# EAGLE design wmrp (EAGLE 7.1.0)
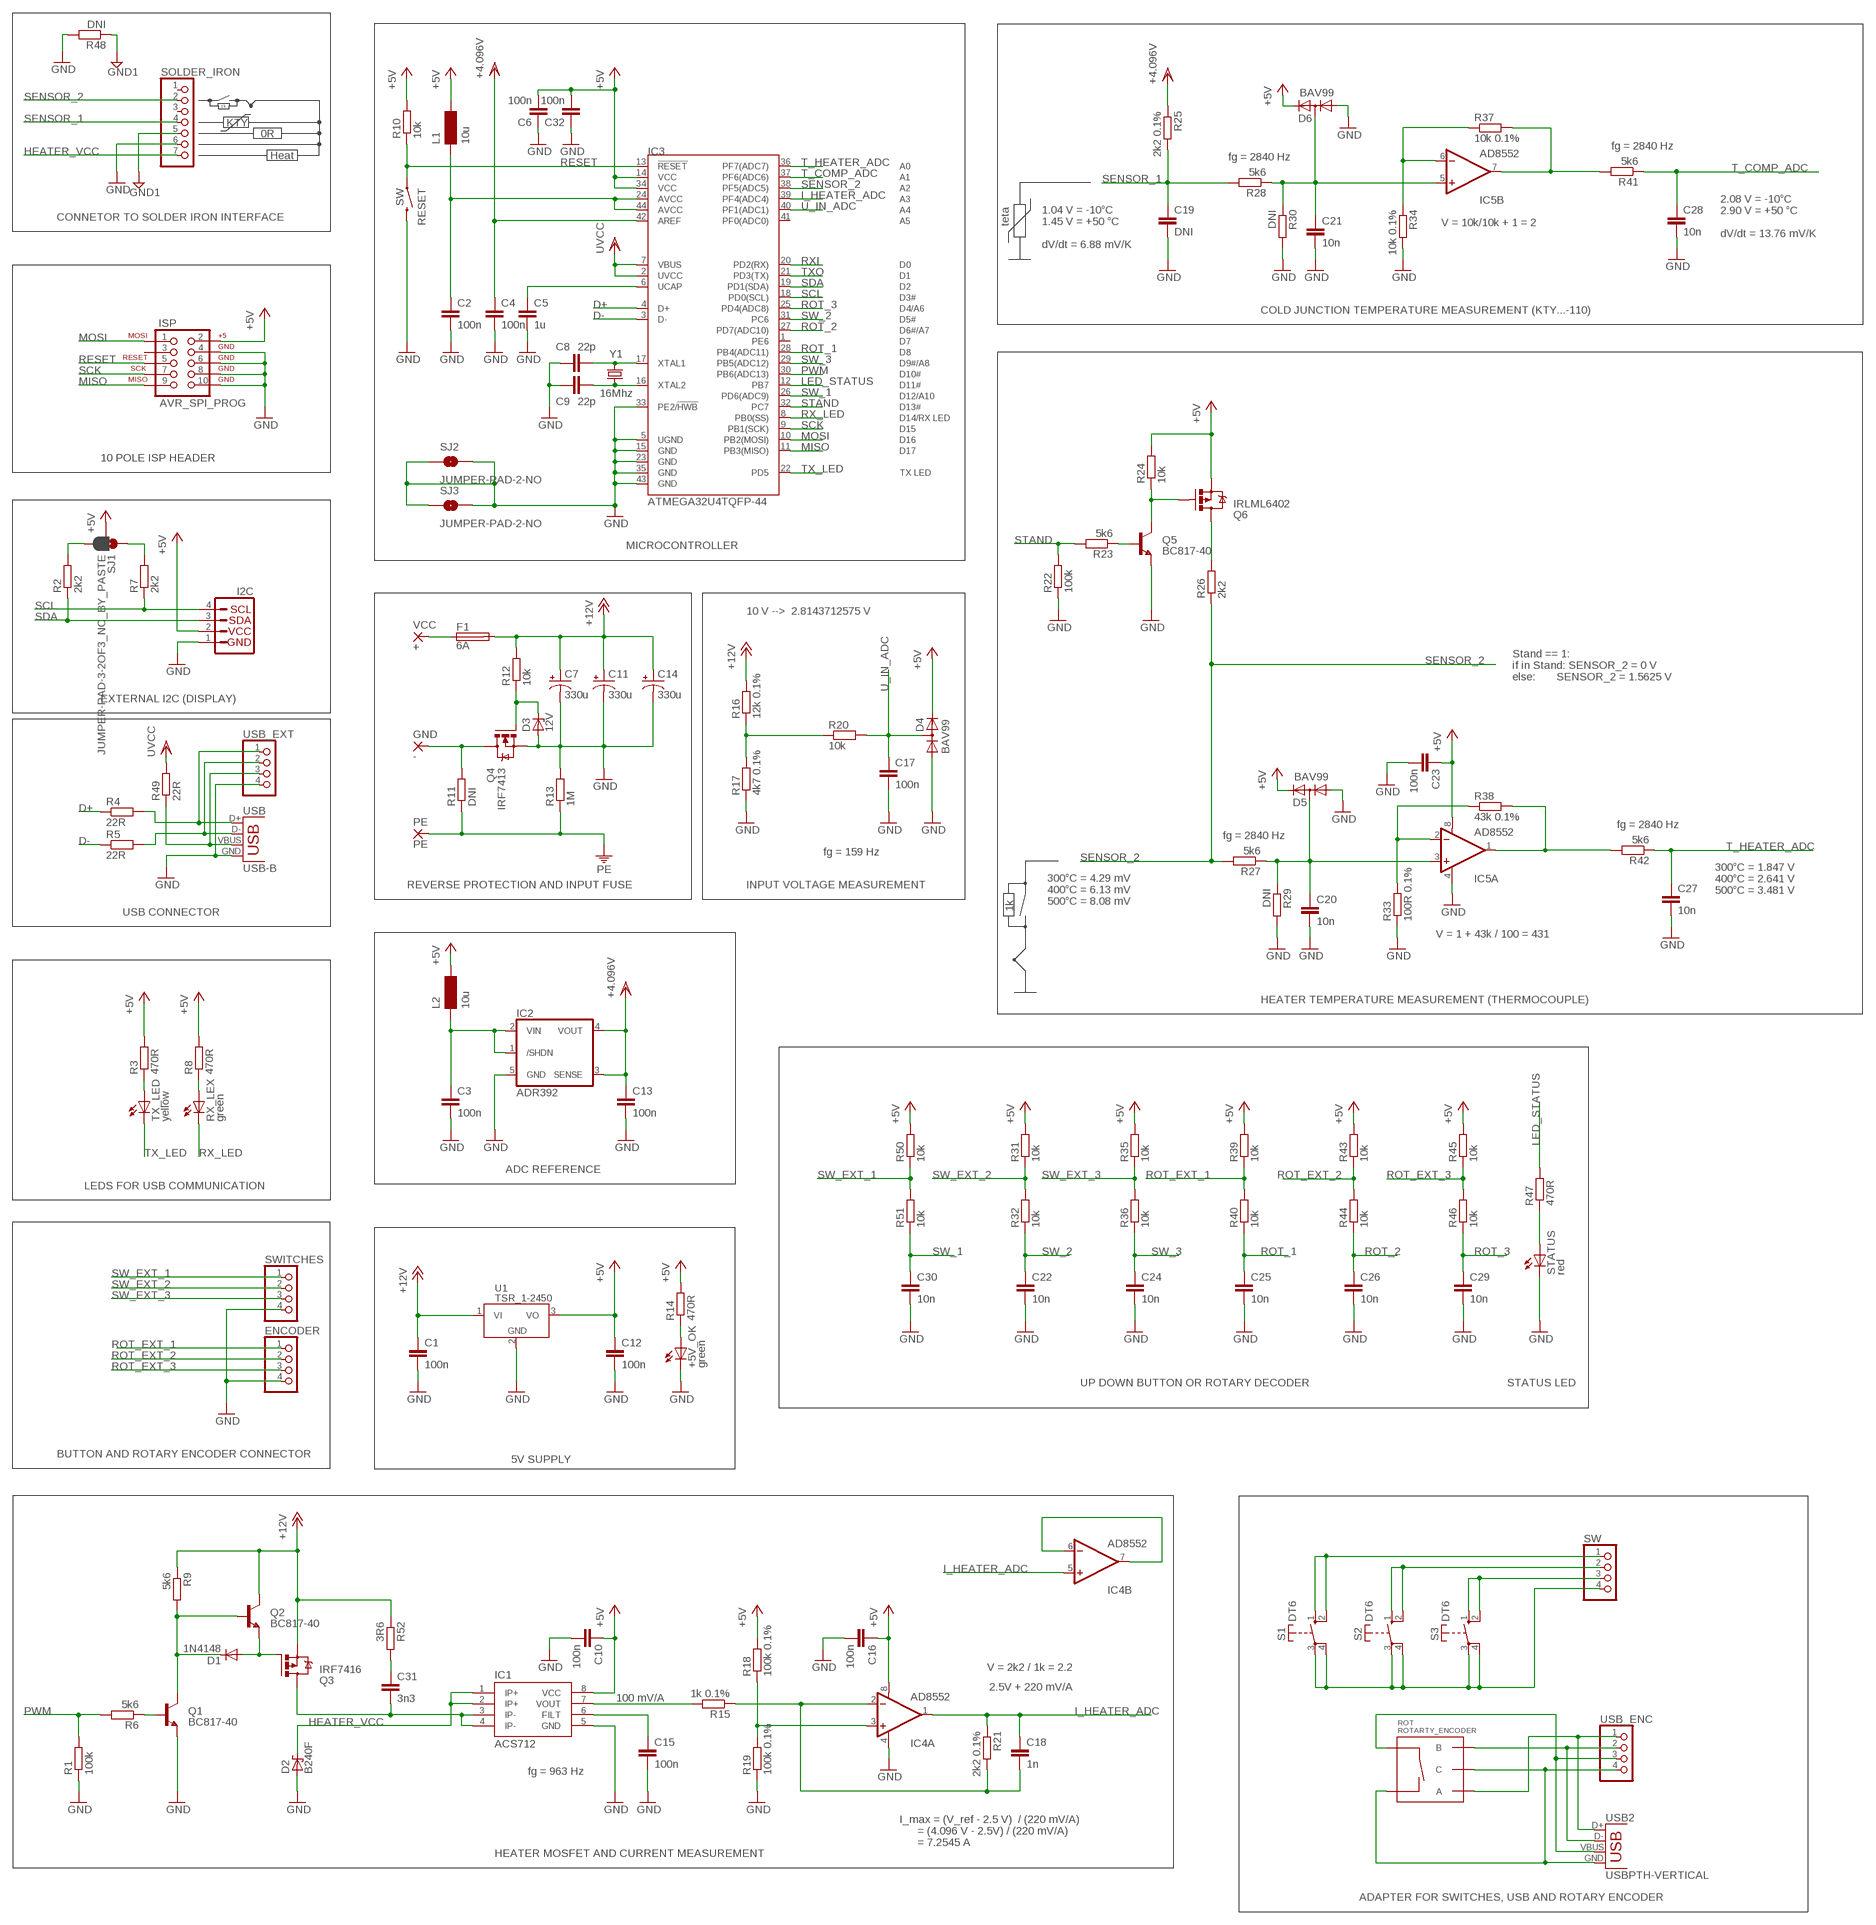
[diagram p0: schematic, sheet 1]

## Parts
+5V_OK  green  LEDCHIPLED_1206  [CHIPLED_1206]
C1  100n  C-EUC1206  [C1206]
C2  100n  C-EUC1206  [C1206]
C3  100n  C-EUC1206  [C1206]
C4  100n  C-EUC1206  [C1206]
C5  1u  C-EUC1206  [C1206]
C6  100n  C-EUC1206  [C1206]
C7  330u  CAP_POLPTH4  [CPOL-RADIAL-1000UF-25V]
C8  22p  C-EUC1206  [C1206]
C9  22p  C-EUC1206  [C1206]
C10  100n  C-EUC1206  [C1206]
C11  330u  CAP_POLPTH4  [CPOL-RADIAL-1000UF-25V]
C12  100n  C-EUC1206  [C1206]
C13  100n  C-EUC1206  [C1206]
C14  330u  CAP_POLPTH4  [CPOL-RADIAL-1000UF-25V]
C15  100n  C-EUC1206  [C1206]
C16  100n  C-EUC1206  [C1206]
C17  100n  C-EUC1206  [C1206]
C18  1n  C-EUC1206  [C1206]
C19  DNI  C-EUC1206  [C1206]
C20  10n  C-EUC1206  [C1206]
C21  10n  C-EUC1206  [C1206]
C22  10n  C-EUC1206  [C1206]
C23  100n  C-EUC1206  [C1206]
C24  10n  C-EUC1206  [C1206]
C25  10n  C-EUC1206  [C1206]
C26  10n  C-EUC1206  [C1206]
C27  10n  C-EUC1206  [C1206]
C28  10n  C-EUC1206  [C1206]
C29  10n  C-EUC1206  [C1206]
C30  10n  C-EUC1206  [C1206]
C31  3n3  C-EUC1206  [C1206]
C32  100n  C-EUC1206  [C1206]
D1  1N4148  DIODE-MINIMELF  [MINIMELF]
D2  B240F  MBRS130LT3  [SMB]
D3  12V  ZENER-DIODESOT23  [SOT23]
D4  BAV99  [SOT23]
D5  BAV99  [SOT23]
D6  BAV99  [SOT23]
ENCODER  PINHD-1X4  [1X04]
F1  6A  SH22,5  [SH22,5]
GND  -  2,54/1,0  [2,2]
I2C  I2C_STANDARD  [1X04]
IC1  ACS712  [SO08]
IC2  ADR392  [SOT23-5]
IC3  ATMEGA32U4TQFP-44  [TQFP44]
IC4  AD8552  OPAMP-DUALU  [SO08]
IC5  AD8552  OPAMP-DUALU  [SO08]
ISP  AVR_SPI_PROG  [AVR_ICSP]
L1  10u  INDUCTOR1206H*  [INDUCTOR-1206]
L2  10u  INDUCTOR1206H*  [INDUCTOR-1206]
PE  PE  2,54/1,0  [2,2]
Q1  BC817-40  TRANSISTOR_NPNSOT23-3  [SOT23-3]
Q2  BC817-40  TRANSISTOR_NPNSOT23-3  [SOT23-3]
Q3  IRF7416  [SO-08]
Q4  IRF7413  [SO-08]
Q5  BC817-40  TRANSISTOR_NPNSOT23-3  [SOT23-3]
Q6  IRLML6402  MOSFET-PCHANNELSMD  [SOT23-3]
R1  100k  R-EU_R1206  [R1206]
R2  2k2  R-EU_R1206  [R1206]
R3  470R  R-EU_R1206  [R1206]
R4  22R  R-EU_R1206  [R1206]
R5  22R  R-EU_R1206  [R1206]
R6  5k6  R-EU_M1206  [M1206]
R7  2k2  R-EU_R1206  [R1206]
R8  470R  R-EU_R1206  [R1206]
R9  5k6  R-EU_M1206  [M1206]
R10  10k  R-EU_R1206  [R1206]
R11  DNI  R-EU_R1206  [R1206]
R12  10k  R-EU_R1206  [R1206]
R13  1M  R-EU_R1206  [R1206]
R14  470R  R-EU_R1206  [R1206]
R15  1k 0.1%  R-EU_M1206  [M1206]
R16  12k 0.1%  R-EU_R1206  [R1206]
R17  4k7 0.1%  R-EU_R1206  [R1206]
R18  100k 0.1%  R-EU_M1206  [M1206]
R19  100k 0.1%  R-EU_M1206  [M1206]
R20  10k  R-EU_R1206  [R1206]
R21  2k2 0.1%  R-EU_M1206  [M1206]
R22  100k  R-EU_R1206  [R1206]
R23  5k6  R-EU_M1206  [M1206]
R24  10k  R-EU_R1206  [R1206]
R25  2k2 0.1%  R-EU_M1206  [M1206]
R26  2k2  R-EU_R1206  [R1206]
R27  5k6  R-EU_M1206  [M1206]
R28  5k6  R-EU_M1206  [M1206]
R29  DNI  R-EU_M1206  [M1206]
R30  DNI  R-EU_M1206  [M1206]
R31  10k  R-EU_R1206  [R1206]
R32  10k  R-EU_R1206  [R1206]
R33  100R 0.1%  R-EU_M1206  [M1206]
R34  10k 0.1%  R-EU_M1206  [M1206]
R35  10k  R-EU_R1206  [R1206]
R36  10k  R-EU_R1206  [R1206]
R37  10k 0.1%  R-EU_M1206  [M1206]
R38  43k 0.1%  R-EU_M1206  [M1206]
R39  10k  R-EU_R1206  [R1206]
R40  10k  R-EU_R1206  [R1206]
R41  5k6  R-EU_M1206  [M1206]
R42  5k6  R-EU_M1206  [M1206]
R43  10k  R-EU_R1206  [R1206]
R44  10k  R-EU_R1206  [R1206]
R45  10k  R-EU_R1206  [R1206]
R46  10k  R-EU_R1206  [R1206]
R47  470R  R-EU_R1206  [R1206]
R48  DNI  R-EU_R1206  [R1206]
R49  22R  R-EU_R1206  [R1206]
R50  10k  R-EU_R1206  [R1206]
R51  10k  R-EU_R1206  [R1206]
R52  3R6  R-EU_M1206  [M1206]
RESET  SW  SWITCH-MOMENTARY-2PTH  [TACTILE-PTH]
ROT  ROTARTY_ENCODER  [ROTARY_ENC_PLAIN]
RX_LEX  green  LEDCHIPLED_1206  [CHIPLED_1206]
S1  DT6  [DT6]
S2  DT6  [DT6]
S3  DT6  [DT6]
SJ1  JUMPER-PAD-3-2OF3_NC_BY_PASTE  [PAD-JUMPER-3-2OF3_NC_BY_PASTE_YES_SILK_FULL_BOX]
SJ2  JUMPER-PAD-2-NO  [PAD-JUMPER-2-NO_NO_SILK]
SJ3  JUMPER-PAD-2-NO  [PAD-JUMPER-2-NO_NO_SILK]
SOLDER_IRON  PINHD-1X7  [1X07]
STATUS  red  LEDCHIPLED_1206  [CHIPLED_1206]
SW  PINHD-1X4  [1X04]
SWITCHES  PINHD-1X4  [1X04]
TX_LED  yellow  LEDCHIPLED_1206  [CHIPLED_1206]
U1  TSR_1-2450  [TSR-1]
USB  USB-B  USBPTH  [USB-B-PTH]
USB2  USBPTH-VERTICAL  [USB-B-PTH-VERTICAL]
USB_ENC  PINHD-1X4  [1X04]
USB_EXT  PINHD-1X4  [1X04]
VCC  +  2,54/1,0  [2,2]
Y1  16Mhz  CRYSTALHC49US  [HC49US]

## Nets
+4.096V: C4.1 C13.1 IC2.3(SENSE) IC2.4(VOUT) IC3.42(AREF) R25.1
+5V: C6.2 C10.1 C12.1 C16.1 C23.1 C32.2 D4.2(C2) D5.2(C2) D6.2(C2) I2C.2 IC1.8(VCC) IC3.14(VCC) IC3.34(VCC) IC4.8(A:V+) IC5.8(A:V+) ISP.2 L1.P$1 L2.P$1 Q6.2(S) R3.2 R8.2 R10.2 R14.2 R18.2 R24.2 R31.2 R35.2 R39.2 R43.2 R45.2 R50.2 SJ1.2 U1.3(VO)
+12V: C1.1 C7.1(+) C11.1(+) C14.1(+) F1.2 Q2.3(C) Q3.1(S) Q3.2(S) Q3.3(S) R9.1 R12.2 R16.2 R52.1 U1.1(VI)
AVCC: C2.1 IC3.24(AVCC) IC3.44(AVCC) L1.P$2
D+: IC3.4(D+) R4.1
D-: IC3.3(D-) R5.1
GND: +5V_OK.C C1.2 C2.2 C3.2 C4.2 C5.2 C6.1 C7.2(-) C8.1 C9.1 C10.2 C11.2(-) C12.2 C13.2 C14.2(-) C15.2 C16.2 C17.2 C19.2 C20.2 C21.2 C22.2 C23.2 C24.2 C25.2 C26.2 C27.2 C28.2 C29.2 C30.2 C32.1 D2.A D3.1(A) D4.1(A1) D5.1(A1) D6.1(A1) ENCODER.4 I2C.1 IC1.5(GND) IC2.5(GND) IC3.5(UGND) IC3.15(GND) IC3.23(GND) IC3.33(PE2/!HWB) IC3.35(GND) IC3.43(GND) IC4.4(A:V-) IC5.4(A:V-) ISP.4 ISP.6 ISP.8 ISP.10 Q1.2(E) Q4.1(S) Q4.2(S) Q4.3(S) Q5.2(E) R1.1 R13.2 R17.1 R19.1 R22.1 R29.2 R30.2 R33.1 R34.2 R48.2 RESET.3 SJ2.1 SJ2.2 SJ3.1 SJ3.2 SOLDER_IRON.6 STATUS.C SWITCHES.4 U1.2(GND) USB.GND USB_EXT.4
GND1: R48.1 SOLDER_IRON.5
HEATER_VCC: D2.C IC1.1(IP+) IC1.2(IP+) SOLDER_IRON.7
I_HEATER_ADC: C18.1 IC3.39(PF4(ADC4)) IC4.1(A:OUT) IC4.5(B:+IN) R21.1
LED_STATUS: IC3.12(PB7) R47.2
MISO: IC3.11(PB3(MISO)) ISP.9
MOSI: IC3.10(PB2(MOSI)) ISP.1
N$1: GND.1(P) Q4.5(D) Q4.6(D) Q4.7(D) Q4.8(D) R11.2
N$2: D3.3(C) Q4.4(G) R12.1
N$3: D1.C Q1.3(C) Q2.1(B) R9.2
N$4: Q1.1(B) R6.1
N$5: F1.1 VCC.1(P)
N$6: R8.1 RX_LEX.A
N$7: S1.3(P) S1.4(P) S2.3(P) S2.4(P) S3.3(P) S3.4(P) SW.4
N$8: S1.1(S) S1.2(S) SW.1
N$9: R4.2 USB.D+ USB_EXT.1
N$10: R5.2 USB.D- USB_EXT.2
N$11: R16.1 R17.2 R20.1
N$12: S2.1(S) S2.2(S) SW.2
N$13: S3.1(S) S3.2(S) SW.3
N$14: R2.2 SJ1.3
N$15: Q5.3(C) Q6.1(G) R24.1
N$16: C15.1 IC1.6(FILT)
N$17: Q5.1(B) R23.1
N$18: IC4.3(A:+IN) R18.1 R19.2
N$19: R3.1 TX_LED.A
N$20: IC1.7(VOUT) R15.2
N$21: C18.2 IC4.2(A:-IN) R15.1 R21.2
N$22: C20.1 D5.3(C1A2) IC5.3(A:+IN) R27.1 R29.1
N$23: Q6.3(D) R26.2
N$24: IC5.2(A:-IN) R33.2 R38.1
N$25: C21.1 D6.3(C1A2) IC5.5(B:+IN) R28.1 R30.1
N$26: D1.A Q2.2(E) Q3.4(G)
N$27: IC5.6(B:-IN) R34.1 R37.1
N$28: C31.2 IC1.3(IP-) IC1.4(IP-) Q3.5(D) Q3.6(D) Q3.7(D) Q3.8(D)
N$29: R7.2 SJ1.1
N$30: C3.1 IC2.1(/SHDN) IC2.2(VIN) L2.P$2
N$31: R49.1 USB.VBUS USB_EXT.3
N$32: R47.1 STATUS.A
N$33: +5V_OK.A R14.1
N$34: IC4.6(B:-IN) IC4.7(B:OUT)
N$39: C31.1 R52.2
N$42: IC5.1(A:OUT) R38.2 R42.2
N$43: IC5.7(B:OUT) R37.2 R41.2
PE: PE.1(P) R11.1 R13.1
PWM: IC3.30(PB6(ADC13)) R1.2 R6.2
RESET: IC3.13(!RESET) ISP.5 R10.1 RESET.1
ROT_1: C25.1 IC3.28(PB4(ADC11)) R40.1
ROT_2: C26.1 IC3.27(PD7(ADC10)) R44.1
ROT_3: C29.1 IC3.25(PD4(ADC8)) R46.1
ROT_A_D+: ROT.A USB2.D+ USB_ENC.1
ROT_B_D-: ROT.B USB2.D- USB_ENC.2
ROT_C_GND: ROT.C ROT.SW- USB2.GND USB_ENC.4
ROT_EXT_1: ENCODER.1 R39.1 R40.2
ROT_EXT_2: ENCODER.2 R43.1 R44.2
ROT_EXT_3: ENCODER.3 R45.1 R46.2
ROT_SW_VBUS: ROT.SW+ USB2.VBUS USB_ENC.3
RX_LED: IC3.8(PB0(SS)) RX_LEX.C
RXI: IC3.20(PD2(RX))
SCK: IC3.9(PB1(SCK)) ISP.7
SCL: I2C.4 IC3.18(PD0(SCL)) R7.1
SDA: I2C.3 IC3.19(PD1(SDA)) R2.1
SENSOR_1: C19.1 R25.2 R28.2 SOLDER_IRON.4
SENSOR_2: IC3.38(PF5(ADC5)) R26.1 R27.2 SOLDER_IRON.2
STAND: IC3.32(PC7) R22.2 R23.2
SW_1: C30.1 IC3.26(PD6(ADC9)) R51.1
SW_2: C22.1 IC3.31(PC6) R32.1
SW_3: C24.1 IC3.29(PB5(ADC12)) R36.1
SW_EXT_1: R50.1 R51.2 SWITCHES.1
SW_EXT_2: R31.1 R32.2 SWITCHES.2
SW_EXT_3: R35.1 R36.2 SWITCHES.3
T_COMP_ADC: C28.1 IC3.37(PF6(ADC6)) R41.1
T_HEATER_ADC: C27.1 IC3.36(PF7(ADC7)) R42.1
TX_LED: IC3.22(PD5) TX_LED.C
TXO: IC3.21(PD3(TX))
U_IN_ADC: C17.1 D4.3(C1A2) IC3.40(PF1(ADC1)) R20.2
UCAP: C5.1 IC3.6(UCAP)
UVCC: IC3.2(UVCC) IC3.7(VBUS) R49.2
XTAL1: C8.2 IC3.17(XTAL1) Y1.2
XTAL2: C9.2 IC3.16(XTAL2) Y1.1
Unconnected: IC3.1(PE6) IC3.41(PF0(ADC0)) ISP.3 SOLDER_IRON.1 SOLDER_IRON.3

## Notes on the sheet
- 1k
- KTY
- 0R
- fg = 2840 Hz
- Heat | fg = 2840 Hz
- CONNETOR TO SOLDER IRON INTERFACE
- teta | V = 10k/10k + 1 = 2
- 2.08 V = -10°C
  2.90 V = +50 °C
  
  dV/dt = 13.76 mV/K
- 1.04 V = -10°C
  1.45 V = +50 °C
  
  dV/dt = 6.88 mV/K
- COLD JUNCTION TEMPERATURE MEASUREMENT (KTY...-110)
- 10 POLE ISP HEADER
- MICROCONTROLLER
- 10 V -->  2.8143712575 V
- Stand == 1:
  if in Stand: SENSOR_2 = 0 V
  else:       SENSOR_2 = 1.5625 V
- EXTERNAL I2C (DISPLAY)
- fg = 2840 Hz
- fg = 2840 Hz
- fg = 159 Hz
- REVERSE PROTECTION AND INPUT FUSE | INPUT VOLTAGE MEASUREMENT
- 300°C = 1.847 V
  400°C = 2.641 V
  500°C = 3.481 V
- 300°C = 4.29 mV
  400°C = 6.13 mV
  500°C = 8.08 mV
- 1k
- USB CONNECTOR
- V = 1 + 43k / 100 = 431
- HEATER TEMPERATURE MEASUREMENT (THERMOCOUPLE)
- ADC REFERENCE
- LEDS FOR USB COMMUNICATION
- UP DOWN BUTTON OR ROTARY DECODER | STATUS LED
- BUTTON AND ROTARY ENCODER CONNECTOR
- 5V SUPPLY
- V = 2k2 / 1k = 2.2
- 2.5V + 220 mV/A
- 100 mV/A
- fg = 963 Hz
- I_max = (V_ref - 2.5 V)  / (220 mV/A)
        = (4.096 V - 2.5V) / (220 mV/A)
        = 7.2545 A
- HEATER MOSFET AND CURRENT MEASUREMENT
- ADAPTER FOR SWITCHES, USB AND ROTARY ENCODER

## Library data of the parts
+5V_OK RX_LEX = led:LED: LED; REICHELT: SMD-LED 1206 GN
C1-C4 C6 C12 C13 C17 C32 = resistor:C-EU: CAPACITOR, European symbol; REICHELT: X7R-G1206 100N
C5 = resistor:C-EU: CAPACITOR, European symbol; REICHELT: X7R-G1206 1,0/50
C7 C11 C14 = SparkFun-Passives:CAP_POL: Capacitor Polarized; REICHELT: RAD FC 330/25
C8 C9 = resistor:C-EU: CAPACITOR, European symbol; REICHELT: NPO-G1206 22P
C10 C15 C16 C23 = rcl:C-EU: CAPACITOR, European symbol; REICHELT: X7R-G1206 100N
C18 = rcl:C-EU: CAPACITOR, European symbol; REICHELT: NPO-G1206 1,0N
C19 = rcl:C-EU: CAPACITOR, European symbol; REICHELT: -
C20-C22 C24-C30 = rcl:C-EU: CAPACITOR, European symbol; REICHELT: X7R-G1206 10N
C31 = resistor:C-EU: CAPACITOR, European symbol; REICHELT: X7R-G1206 3,3N
D1 = diode:DIODE-: DIODE; REICHELT: 1N 4148 SMD
D2 = diode:MBRS130LT3: Schottky Power Rectifier; REICHELT: B 240 F
D3 = diode:ZENER-DIODE: Z-Diode; REICHELT: SMD ZD 12
D4-D6 = BAV99:BAV99: Small Signal Diode Source: http://www.fairchildsemi.com/ds/BA/BAV99.pdf; REICHELT: BAV 99 SMD
ENCODER SW SWITCHES USB_ENC USB_EXT = pinhead:PINHD-1X4: PIN HEADER; REICHELT: MPE 087-1-004
F1 = fuse:SH22,5: FUSE HOLDER; MF: SCHURTER; MPN: 0031.8201; OC_FARNELL: 1162740; OC_NEWARK: 96F8317; REICHELT: PL OGN-22,5
GND PE VCC = WIREPAD22:2,54/1,0: THROUGH-HOLE PAD; REICHELT: -
I2C = SparkFun-Connectors:I2C_STANDARD: SparkFun has standardized on a pinout for all I2C based sensor breakouts. This pinout allows I2C boards to be plugged directly into the headers on Arduino Uno compatible boards, and to be daisy chained easily.; REICHELT: MPE 087-1-004
IC1 = SparkFun-AnalogIC:ACS712: Hall-effect-based isolated linear current sensor
IC2 = wmrp:ADR392: http://www.analog.com/media/en/technical-documentation/data-sheets/ADR391_392_395.pdf; CONRAD: 1250814 - 62; VOELKNER: A376911
IC3 = SparkFun-DigitalIC:ATMEGA32U4: Atmel 44-pin 8-bit Microcontroller with 32KBytes of ISP Flash and USB Controller; VOELKNER: A886841
IC4 IC5 = SparkFun-AnalogIC:OPAMP-DUAL: Generic op-amp footprint; REICHELT: AD 8552 AR
ISP = SparkFun-Connectors:AVR_SPI_PROG: AVR 10-pin ICSP Header This is the standard AVR In Circuit Serial Programming header. Minimal, but includes pin one indicator. Works with standard Olimex programmers. Also look for the 6-pin reduced version. Spark Fun Electronics SKU: PRT-00778; REICHELT: MPE 087-2-010
L1 L2 = wmrp:INDUCTOR: Inductors; REICHELT: L-1812AF 10µ
Q1 Q2 Q5 = SparkFun-DiscreteSemi:TRANSISTOR_NPN: Generic NPN BJT MMBT2222A - TRANS-08049 (SOT-23, 1A 40V) MPSA42 - TRANS-09116 (SOT-23, 500mA 300V) MMBT5088LT1G - TRANS-11160 (SOT-23, 50 mA 30V) BC547 - COM-08928 (TO-92 45V 100mA) (1.Collector 2.Base 3.Emitter) 2N3904 - COM-00521 (TO-92 40V 200mA) (1.Emitter 2.Base 3.Collector) P2N2222A -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; PROD_ID: TRANS-08049; REICHELT: BC 817-40 SMD
Q3 = wmrp:IRF7416: P-Channel HEXFET® Power MOSFET http://www.irf.com/product-info/datasheets/data/irf7416.pdf; REICHELT: IRF 7416
Q4 = wmrp:IRF7413: N-Channel HEXFET® Power MOSFET http://www.irf.com/product-info/datasheets/data/irf7413.pdf; REICHELT: IRF 7413
Q6 = SparkFun-DiscreteSemi:MOSFET-PCHANNEL: Generic PMOSFET IRLML2244 - TRANS-11153 (SOT-23 -20V -4.3A) (1.Gate 2.Source 3.Drain) FQP27P06 - COM-10349 (TO-220 -60V -27A) (1.Gate 2.Source 3.Drain); REICHELT: IRLML 6402
R1 R22 = resistor:R-EU_: RESISTOR, European symbol; REICHELT: SMD 1/4W 100K
R2 R7 R26 = resistor:R-EU_: RESISTOR, European symbol; REICHELT: SMD 1/4W 2,2K
R3 R8 R14 R47 = resistor:R-EU_: RESISTOR, European symbol; REICHELT: SMD 1/4W 470
R4 R5 R49 = resistor:R-EU_: RESISTOR, European symbol; REICHELT: SMD 1/4W 22
R6 R9 R23 R27 R28 R41 R42 = rcl:R-EU_: RESISTOR, European symbol; REICHELT: SMD 1/4W 5,6K
R10 R12 R20 R24 R31 R32 R35 R36 R39 R40 R43-R46 R50 R51 = resistor:R-EU_: RESISTOR, European symbol; REICHELT: SMD 1/4W 10K
R11 R48 = resistor:R-EU_: RESISTOR, European symbol; REICHELT: -
R13 = resistor:R-EU_: RESISTOR, European symbol; REICHELT: SMD 1/4W 1,0M
R15 = rcl:R-EU_: RESISTOR, European symbol; REICHELT: SPR-1206 1,00K
R16 = resistor:R-EU_: RESISTOR, European symbol; REICHELT: SPR-1206 12,0K
R17 = resistor:R-EU_: RESISTOR, European symbol; REICHELT: SPR-1206 4,70K
R18 R19 = rcl:R-EU_: RESISTOR, European symbol; REICHELT: SPR-1206 100K
R21 R25 = rcl:R-EU_: RESISTOR, European symbol; REICHELT: SPR-1206 2,20K
R29 R30 = rcl:R-EU_: RESISTOR, European symbol; REICHELT: -
R33 = rcl:R-EU_: RESISTOR, European symbol; REICHELT: SPR-1206 100
R34 R37 = rcl:R-EU_: RESISTOR, European symbol; REICHELT: SPR-1206 10,0K
R38 = rcl:R-EU_: RESISTOR, European symbol; REICHELT: SPR-1206 43,0K
R52 = rcl:R-EU_: RESISTOR, European symbol; REICHELT: SMD 1/4W 3,6
RESET = SparkFun-Electromechanical:SWITCH-MOMENTARY-2: Various NO switches- pushbuttons, reed, etc; REICHELT: TASTER 9302
ROT = SparkFun-Electromechanical:ROTARTY_ENCODER: Simple no LED rotary encoder Example: COM-09117; VOELKNER: W32173
S1-S3 = switch-misc:DT: ITT SWITCH; VOELKNER: D76189
SJ1 = SparkFun-Passives:JUMPER-PAD-3-2OF3_NC_BY_PASTE; REICHELT: -
SJ2 SJ3 = SparkFun-Passives:JUMPER-PAD-2-NO; REICHELT: -
SOLDER_IRON = pinhead:PINHD-1X7: PIN HEADER; REICHELT: -
STATUS = led:LED: LED; REICHELT: SMD-LED 1206 RT
TX_LED = led:LED: LED; REICHELT: SMD-LED 1206 GE
U1 = traco_tsr-1:TSR_1-*; REICHELT: TSR 1-2450
USB = SparkFun-Connectors:USB: USB Connectors USB-B-PTH is fully proven SKU : PRT-00139/CONN-08278 USB-miniB is fully proven SKU : PRT-00587 USB-A-PCB is untested. USB-A-H is throughly reviewed, but untested. Spark Fun Electronics SKU : PRT-00437 USB-B-SMT is throughly reviewed, but untested. Needs silkscreen touching up.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; PROD_ID: CONN-08278; REICHELT: USB BW
USB2 = wmrp:USB: USB Connectors USB-B-PTH is fully proven SKU : PRT-00139/CONN-08278 USB-miniB is fully proven SKU : PRT-00587 USB-A-PCB is untested. USB-A-H is throughly reviewed, but untested. Spark Fun Electronics SKU : PRT-00437 USB-B-SMT is throughly reviewed, but untested. Needs silkscreen touching up.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; REICHELT: USB BG
Y1 = SparkFun-FreqCtrl:CRYSTAL: Various standard crystals. Proven footprints.; REICHELT: 16,0000-HC49U-S

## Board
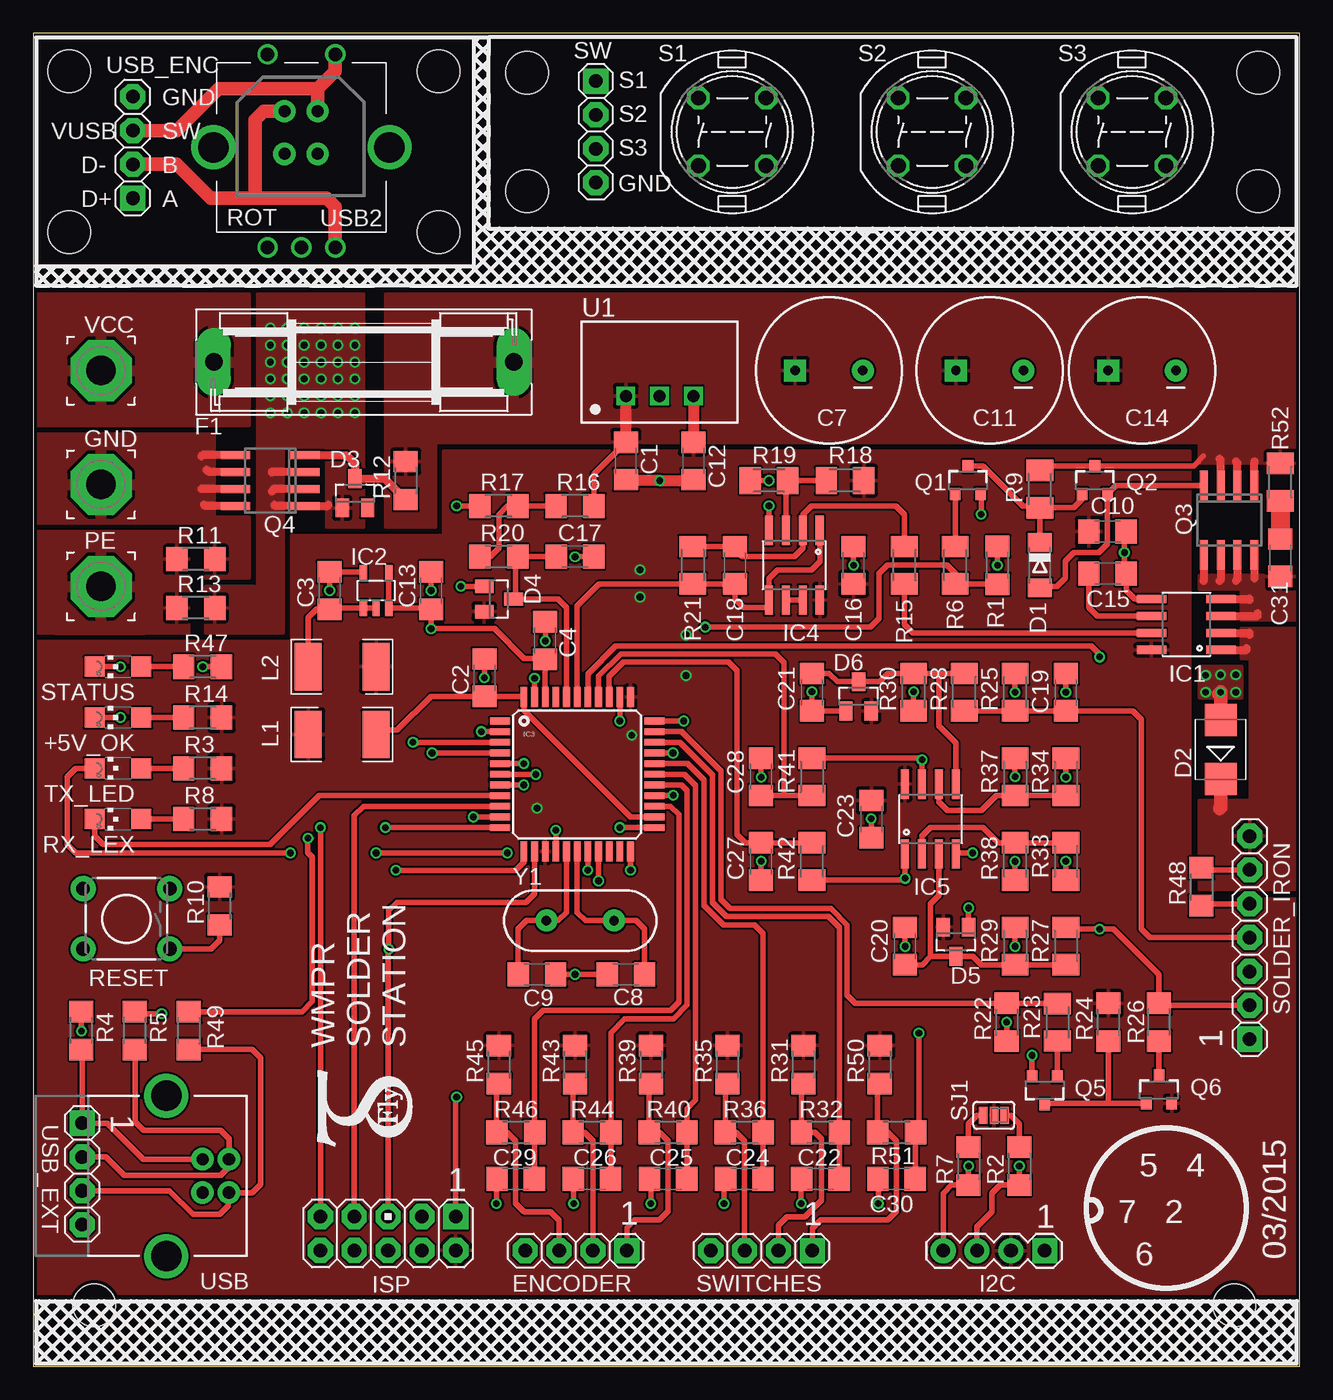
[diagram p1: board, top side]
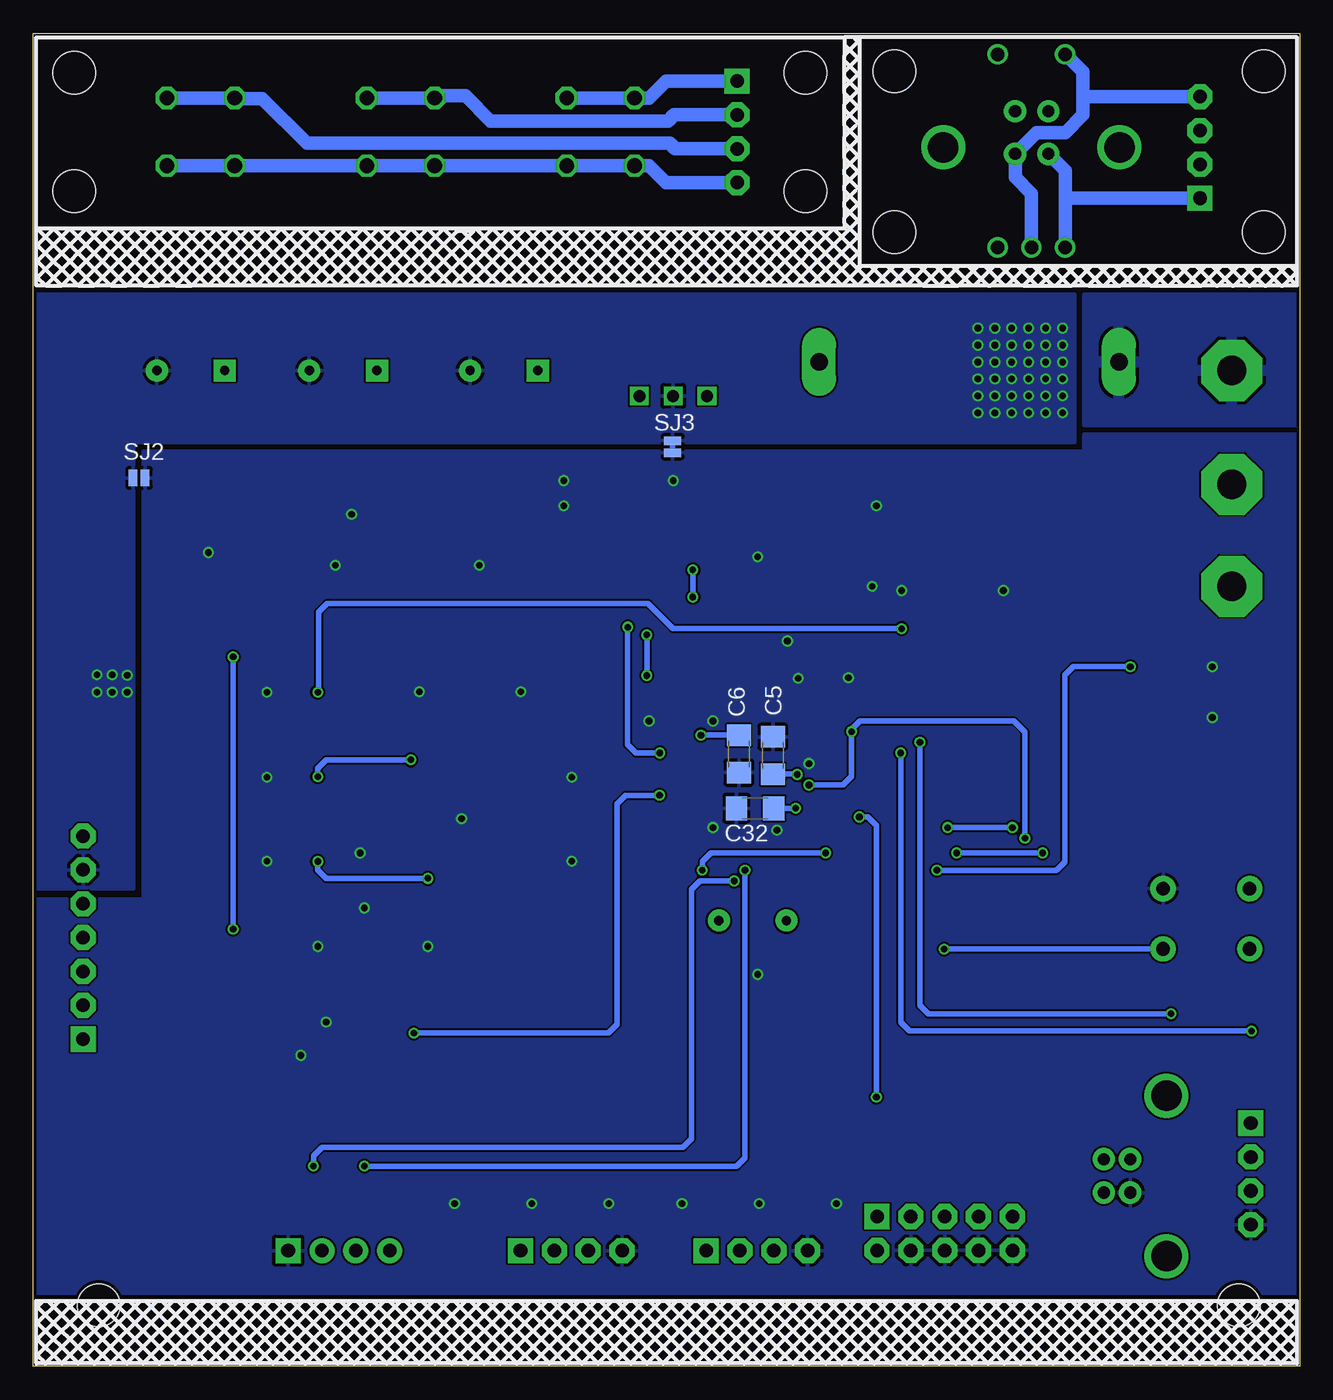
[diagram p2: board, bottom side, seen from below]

Size 95 x 100 mm. Coordinates in mm from the lower left corner, seen from the top.
Outline: 0,0 95,0 95,100 0,100 0,0
Copper layers (1*16): Top 0.035mm / dielectric 1.5mm / Bottom 0.035mm
Design rules "Elecrow_2-layer_eagle_rule": minimum track width 6mil, minimum drill 12mil, track to track 6mil, track to pad 6mil, pad to pad 6mil, via to via 6mil, smd to smd 0mil, copper to edge 10mil, drill to drill 10mil, minimum pad ring 10mil, minimum via ring 6mil, stop-mask expansion 2mil, vias tented up to drill 100mil, thermal gap 10mil
Holes 3.2 mm at 37.06,97.05 2.68,97.16 90.09,4.57 4.57,4.57 91.92,97.05 30.4,97.16 37.06,88.16 30.4,85.09 2.68,85.09 91.92,88.16

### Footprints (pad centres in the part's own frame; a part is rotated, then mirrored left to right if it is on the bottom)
CHIPLED_1206 = smd 1.5 x 1.5: A 0,-1.75; C 0,1.75
C1206 = smd 1.6 x 1.8: 1 -1.4,0; 2 1.4,0
CPOL-RADIAL-1000UF-25V = drill 0.7 pad 1.651 square: 1 2.54,0 | drill 0.7 pad 1.651: 2 -2.54,0
MINIMELF = smd 1.4 x 1.8: A 1.7,0; C -1.7,0
SMB = smd 2.4 x 2.4: A 2.2,0; C -2.2,0
SOT23 = smd 1 x 1.4: 1 -0.95,-1.1; 2 0.95,-1.1; 3 0,1.1
1X04 = drill 1.016 pad 1.88 square: 1 -3.81,0 | drill 1.016 pad 1.88 octagon: 2 -1.27,0; 3 1.27,0; 4 3.81,0
SH22,5 = drill 1.321 pad 2.54 long: 1 -11.252,0; 2 11.252,0
2,2 = drill 2.2 pad 4.572 octagon: 1 0,0
1X04' = drill 1.016 pad 1.88 square: 1 0,0 | drill 1.016 pad 1.88: 2 2.54,0; 3 5.08,0; 4 7.62,0
SO08 = smd 0.61 x 2.21: 1 -1.905,-2.616; 2 -0.635,-2.616; 3 0.635,-2.616; 4 1.905,-2.616; 5 1.905,2.616; 6 0.635,2.616; 7 -0.635,2.616; 8 -1.905,2.616
SOT23-5 = smd 0.55 x 1.2: 1 -0.95,-1.3; 2 0,-1.3; 3 0.95,-1.3; 4 0.95,1.3; 5 -0.95,1.3
TQFP44 = smd 1.5 x 0.5: 1 -5.8,4; 2 -5.8,3.2; 3 -5.8,2.4; 4 -5.8,1.6; 5 -5.8,0.8; 6 -5.8,0; 7 -5.8,-0.8; 8 -5.8,-1.6; 9 -5.8,-2.4; 10 -5.8,-3.2; 11 -5.8,-4; 23 5.8,-4; 24 5.8,-3.2; 25 5.8,-2.4; 26 5.8,-1.6; 27 5.8,-0.8; 28 5.8,0; 29 5.8,0.8; 30 5.8,1.6; 31 5.8,2.4; 32 5.8,3.2; 33 5.8,4 | smd 0.5 x 1.5: 12 -4,-5.8; 13 -3.2,-5.8; 14 -2.4,-5.8; 15 -1.6,-5.8; 16 -0.8,-5.8; 17 0,-5.8; 18 0.8,-5.8; 19 1.6,-5.8; 20 2.4,-5.8; 21 3.2,-5.8; 22 4,-5.8; 34 4,5.8; 35 3.2,5.8; 36 2.4,5.8; 37 1.6,5.8; 38 0.8,5.8; 39 0,5.8; 40 -0.8,5.8; 41 -1.6,5.8; 42 -2.4,5.8; 43 -3.2,5.8; 44 -4,5.8
AVR_ICSP = drill 1.016 pad 1.88 square: 1 -1.27,5.08 | drill 1.016 pad 1.88 octagon: 2 1.27,5.08; 3 -1.27,2.54; 4 1.27,2.54; 5 -1.27,0; 6 1.27,0; 7 -1.27,-2.54; 8 1.27,-2.54; 9 -1.27,-5.08; 10 1.27,-5.08
INDUCTOR-1206 = smd 2.032 x 3.556: P$1 -2.54,0; P$2 2.54,0
SOT23-3 = smd 0.8 x 0.9: 1 -0.95,-1; 2 0.95,-1; 3 0,1.1
SO-08 = smd 0.6 x 2.2: 1 -1.905,-2.6; 2 -0.635,-2.6; 3 0.635,-2.6; 4 1.905,-2.6; 5 1.905,2.6; 6 0.635,2.6; 7 -0.635,2.6; 8 -1.905,2.6
R1206 = smd 1.6 x 1.803: 1 -1.422,0; 2 1.422,0
M1206 = smd 1.6 x 2: 1 -1.4,0; 2 1.4,0
TACTILE-PTH = drill 1.016 pad 1.88: 1 -3.251,2.261; 2 3.251,2.261; 3 -3.251,-2.261; 4 3.251,-2.261
ROTARY_ENC_PLAIN = drill 1.016: A 7.493,-2.54; B 7.493,2.54; C 7.493,0; SW+ -6.985,2.54; SW- -6.985,-2.54 | drill 2.286: P$3 0,6.604; P$4 0,-6.604
DT6 = drill 1.118 octagon: 1 -2.54,2.54; 2 2.54,2.54; 3 2.54,-2.54; 4 -2.54,-2.54
PAD-JUMPER-3-2OF3_NC_BY_PASTE_YES_SILK_FULL_BOX = smd 0.635 x 1.27: 1 -0.813,0; 2 0,0; 3 0.813,0
PAD-JUMPER-2-NO_NO_SILK = smd 0.635 x 1.27: 1 -0.45,0; 2 0.45,0
1X07 = drill 1.016 pad 1.88 square: 1 -7.62,0 | drill 1.016 pad 1.88 octagon: 2 -5.08,0; 3 -2.54,0; 4 0,0; 5 2.54,0; 6 5.08,0; 7 7.62,0
TSR-1 = drill 0.9 square: 1 -2.54,0; 2 0,0; 3 2.54,0
USB-B-PTH = drill 0.914 pad 1.676: D+ 0,1.25; D- 1.981,1.25; GND 0,-1.25; VBUS 1.981,-1.25 | drill 2.286: S1 -2.718,-6.02; S2 -2.718,6.02
USB-B-PTH-VERTICAL = drill 0.914 pad 1.676: D+ 4.826,4.394; D- 4.826,7.595; GND 7.315,4.394; VBUS 7.315,7.595
HC49US = drill 0.7 pad 1.651: 1 -2.54,0; 2 2.54,0

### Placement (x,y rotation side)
+5V_OK  6.35,48.67 90 top
C1  44.45,67.92 270 top
C2  33.85,51.65 90 top
C3  22.23,58.19 90 top
C4  38.39,54.44 90 top
C5  39.51,45.82 90 bottom
C6  42.06,45.94 90 bottom
C7  59.69,74.7 180 top
C8  44.45,29.39 0 top
C9  37.78,29.39 180 top
C10  80.59,62.64 0 top
C11  71.75,74.7 180 top
C12  49.53,67.92 270 top
C13  29.84,58.19 90 top
C14  83.19,74.7 180 top
C15  80.59,59.46 0 top
C16  61.54,60.1 90 top
C17  40.64,60.73 0 top
C18  52.65,60.1 90 top
C19  77.47,50.57 90 top
C20  65.41,31.52 90 top
C21  58.42,50.57 270 top
C22  59.05,14.06 180 top
C23  62.87,41.05 270 top
C24  53.34,14.06 180 top
C25  47.62,14.06 180 top
C26  41.91,14.06 180 top
C27  54.61,37.87 270 top
C28  54.61,44.22 90 top
C29  36.2,14.06 180 top
C30  64.77,14.06 180 top
C31  93.56,60.66 270 top
C32  40.84,41.86 0 bottom
D1  75.51,60.1 270 top
D2  89.08,46.27 90 top
D3  24.13,65.49 0 top
D4  34.92,57.56 270 top
D5  69.22,31.84 180 top
D6  61.91,50.25 0 top
ENCODER  40.72,8.66 180 top
F1  24.79,75.34 0 top
GND  5.08,66.15 0 top
I2C  [1X04']  75.88,8.66 180 top
IC1  86.51,55.65 90 top
IC2  25.72,58.19 0 top
IC3  40.81,44.41 0 top
IC4  57.1,60.1 180 top
IC5  67.31,41.05 0 top
ISP  26.62,9.96 270 top
L1  23.16,47.4 0 top
L2  23.16,52.48 180 top
PE  5.08,58.51 0 top
Q1  70.12,66.45 0 top
Q2  79.64,66.45 0 top
Q3  89.71,63.49 180 top
Q4  17.78,66.45 90 top
Q5  75.88,20.73 180 top
Q6  84.45,20.73 0 top
R1  72.34,60.1 270 top
R2  73.98,15.01 90 top
R3  12.7,44.86 0 top
R4  3.61,25.17 270 top
R5  7.62,25.17 270 top
R6  69.16,60.1 270 top
R7  70.17,15.01 90 top
R8  12.7,41.05 0 top
R9  75.51,65.81 270 top
R10  13.97,34.53 90 top
R11  12.19,60.55 0 top
R12  27.94,66.45 90 top
R13  12.19,56.9 0 top
R14  12.7,48.67 0 top
R15  65.35,60.1 270 top
R16  40.64,64.54 0 top
R17  34.92,64.54 0 top
R18  60.91,66.45 0 top
R19  55.19,66.45 0 top
R20  34.92,60.73 0 top
R21  49.48,60.1 90 top
R22  73.03,25.81 90 top
R23  76.83,25.81 90 top
R24  80.64,25.81 90 top
R25  73.66,50.57 270 top
R26  84.45,25.81 270 top
R27  77.47,31.52 90 top
R28  69.85,50.57 270 top
R29  73.66,31.52 90 top
R30  66.04,50.57 270 top
R31  57.78,22.63 90 top
R32  59.05,17.55 180 top
R33  77.47,37.87 90 top
R34  77.47,44.22 90 top
R35  52.07,22.63 90 top
R36  53.34,17.55 180 top
R37  73.66,44.22 90 top
R38  73.66,37.87 270 top
R39  46.35,22.63 90 top
R40  47.62,17.55 180 top
R41  58.42,44.22 90 top
R42  58.42,37.87 270 top
R43  40.64,22.63 90 top
R44  41.91,17.55 180 top
R45  34.92,22.63 90 top
R46  36.2,17.55 180 top
R47  12.7,52.48 0 top
R48  87.63,35.97 90 top
R49  11.66,25.17 90 top
R50  63.5,22.63 90 top
R51  64.77,17.55 180 top
R52  93.56,66.33 270 top
RESET  6.99,33.57 180 top
ROT  20.12,91.44 270 top
RX_LEX  6.35,41.05 90 top
S1  52.44,92.61 0 top
S2  67.44,92.61 0 top
S3  82.44,92.61 0 top
SJ1  72.07,18.82 0 top
SJ2  87.07,66.65 180 bottom
SJ3  47.04,68.99 90 bottom
SOLDER_IRON  91.26,32.16 90 top
STATUS  6.35,52.48 90 top
SW  42.2,92.61 270 top
SWITCHES  54.64,8.66 180 top
TX_LED  6.35,44.86 90 top
U1  46.99,72.8 0 top
U$1  [LOGO+]  28.57,15.65 90 top
USB  12.7,14.27 0 top
USB2  14.02,86.56 0 top
USB_ENC  7.47,91.44 90 top
USB_EXT  3.66,14.43 270 top
VCC  5.08,74.7 0 top
Y1  41.03,33.43 0 top

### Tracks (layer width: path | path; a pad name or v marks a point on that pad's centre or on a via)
+4.096V  (via drill 0.5 pad 0.3)
  Top 0.406: IC2.4 IC2.3 29.84,56.89 C13.1 v29.84,55.33 34.61,55.33 36.83,53.11 38.39,53.11 C4.1 38.41,53.05 IC3.42 | R25.1 v73.66,50.57
  Bottom 0.406: v29.84,55.33 47.02,55.33 48.9,57.21 72.97,57.21 73.61,56.58 73.61,50.57 v73.66,50.57
+5V  (via drill 0.5 pad 0.25, 0.5 pad 0.3)
  Top 0.406: IC3.34
  Top 0.813: U1.3 C12.1
  Bottom 0.406: C6.2 42.07,47.35 v44.91,47.35 | C32.2 v37.8,41.86 | v48.97,54.86 48.97,51.61 | v45.52,57.71 v45.52,59.74
  other vias: 48.97,51.82
  pour Top: 0,54.38 19.37,54.38 19.37,62.32 30.8,62.32 30.8,68.67 86.78,68.67 86.78,58.42 86.77,58.42 86.77,52.83 86.78,35.04 94.78,35.04 94.78,5.49 -0.03,5.49
+12V
  Top 0.406: R9.1 75.51,67.55 Q2.3 87.05,67.55 87.78,68.28 | C1.1 42.06,66.93 R16.2
  Top 0.61: Q3.3 89.08,68 89,68.07 | Q3.2 90.35,67.74 90.22,67.87 | Q3.1 91.62,67.84 91.64,67.87
  Top 0.813: C1.1 U1.1
  pour Top: 26.44,80.42 26.44,62.95 30.16,62.95 30.16,69.3 94.78,69.3 94.78,80.42
  pour Top: 87.46,67.74 94.78,67.74 94.78,70.89 87.46,70.89
  pour Top: 32.72,78.84 32.72,71.32 39.22,71.32 39.22,78.84
AVCC
  Top 0.406: L1.P$2 25.7,47.71 27.3,47.71 29.84,50.25 C2.1 36.76,50.25 IC3.44 36.8,49.21 44.81,41.21 IC3.24 | IC3.24
D+  (via drill 0.5 pad 0.3)
  Top 0.406: R4.1 v3.61,25.15 | IC3.4 | IC3.4 v29.92,46.01
  Bottom 0.406: v3.61,25.15 29.29,25.15 29.92,25.78 v29.92,46.01
D-  (via drill 0.5 pad 0.3)
  Top 0.406: R5.1 7.62,26.44 v9.64,26.44 | IC3.3 | IC3.3 v28.49,46.81
  Bottom 0.406: v28.49,46.81 28.49,27.08 27.85,26.44 v9.64,26.44
GND  (via drill 0.5 pad 0.3)
  Top 0.406: IC2.5 24.77,59.59 C3.2 v22.23,58.19 | C13.2 v29.84,58.19 | R17.1 v31.75,64.54 | C17.2 v40.64,60.73 | D4.1 arc90 D4.1 v32.07,58.51 | STATUS.C v6.54,52.48 | +5V_OK.C v6.54,48.67 | v72.34,60.1 R1.1 | IC1.5 82.63,57.56 81.99,58.19 C15.2 81.86,59.46 v81.86,61.05 81.86,62.64 C10.2 | v55.19,66.45 R19.1 arc-90 53.92,66.32 | C16.2 v61.54,60.1 | IC4.4 v55.19,64.54 | C25.2 46.23,13.74 46.35,13.74 46.33,13.72 v46.33,12.19 | 70.17,32.92 D5.1 v70.17,34.38 | R29.2 v73.66,31.5 | C20.2 v65.41,31.5 | R33.1 v77.47,37.9 | R34.2 v77.47,44.2 | R30.2 v66.04,50.6 | D6.1 60.96,49.17 C21.2 v58.42,50.6 | C28.2 v54.61,44.2 | C27.2 v54.61,37.9 | C23.2 v62.87,41.07 | IC5.4 69.22,38.51 v70.48,38.51 | C9.1 v40.64,29.39 C8.1 | IC3.35 v44.01,48.41 | v44.01,48.41 | IC3.33 | IC3.5 | IC3.5 v36.8,45.21 | IC3.15 v39.2,40.21 | v39.2,40.21 | IC3.23 v44.01,40.41 | C4.2 38.42,55.84 v38.42,54.41 | IC3.43 | IC3.43 v37.6,51.61 | IC3.33 v48.81,48.41 | C2.2 v33.85,51.65 | v48.81,48.41 | C19.2 v77.47,50.57 | Q1.2 71.12,65.39 v71.12,63.91 | R22.1 v73.03,25.81 | SOLDER_IRON.6 87.78,37.24 R48.2 | C29.2 34.75,14.01 v34.75,12.19 | C26.2 40.54,14.03 v40.54,12.19 | C24.2 51.82,13.94 v51.82,12.19 | C22.2 57.61,14.01 v57.61,12.19 | C30.2 63.4,14.03 v63.4,12.19 | Q5.2 v74.93,23.31
  Top 0.61: 18.09,64.62 18.16,64.54 Q4.1 22.07,64.54 22.15,64.62 | Q4.2 18.06,65.81 17.88,65.63 | Q4.3 17.91,67.08 17.88,67.06
  Top 0.813: C1.2 44.45,66.45 v46.99,66.45 49.53,66.45 C12.2
  Top 1.016: 88.95,50.44 v89.08,50.57 D2.A
  Top 1.27: D2.A 88.95,48.47
  Bottom 0.406: SJ3.1 SJ3.2
  other vias: 17.78,77.88 87.96,50.57 90.22,50.57 89.08,51.87 87.96,51.84 19.05,77.88 20.32,77.88 20.32,76.61 19.05,76.61 17.78,76.61 17.78,75.34 19.05,75.34 20.32,75.34 20.32,74.07 19.05,74.07 17.78,74.07 17.78,72.8 19.05,72.8 20.32,72.8 20.32,71.53 19.05,71.53 17.78,71.53 90.22,51.87 21.59,77.88 21.59,76.61 21.59,75.34 21.59,74.07 21.59,72.8 21.59,71.53 22.86,71.53 22.86,72.8 22.86,74.07 22.86,75.34 22.86,76.61 22.86,77.88 24.13,71.53 24.13,72.8 24.13,74.07 24.13,75.34 24.13,76.61 24.13,77.88
  pour Bottom: 0.09,69.94 16.19,69.94 16.19,68.67 86.77,68.67 86.77,35.04 94.78,35.04 94.78,5.49 0,5.49
  pour Bottom: 16.87,80.42 94.78,80.42 94.78,35.79 87.46,35.79 87.46,69.3 16.87,69.3
  pour Top: 16.83,68.95 16.83,80.42 22.3,80.42 22.3,68.95
  pour Top: 22,62.95 24.77,62.95 24.77,80.42 22,80.42
  pour Top: 12.93,55.02 18.73,55.02 18.73,69.39 16.83,69.39 16.83,58.51 12.93,58.51
  pour Top: 87.46,52.48 87.46,50.14 90.65,50.14 90.65,52.48
GND1
  Top 0.406: SOLDER_IRON.5 88.32,34.7 88.16,34.54 R48.1
HEATER_VCC
  Top 0.61: IC1.2 91.24,55.02 91.24,54.86 | IC1.1 91.03,53.75 91.03,53.85
  Top 1.016: D2.C 89.08,41.94 89,41.86
  Top 1.27: D2.C 89,44.07
  pour Top: 90.61,55.33 90.61,53.11 91.29,53.11 91.29,42.44 87.46,42.44 87.46,35.78 94.78,35.78 94.78,55.33
I_HEATER_ADC
  Top 0.406: IC3.39 40.8,57.05 42.46,58.7 R21.1 C18.1 52.65,57.56 53.29,56.92 55.19,56.92 IC4.5 55.19,59.11 55.83,59.74 58.37,59.74 59,60.38 IC4.1
LED_STATUS  (via drill 0.5 pad 0.3)
  Top 0.406: IC3.12 | R47.2 v12.7,52.48 | IC3.12 36.8,37.85 36.17,37.21 v27.2,37.21
  Bottom 0.406: v27.2,37.21 18.24,37.21 17.6,37.85 17.6,51.84 16.97,52.48 v12.7,52.48
MISO  (via drill 0.5 pad 0.3)
  Top 0.406: IC3.11 v26.4,40.41 | v21.54,40.41 ISP.9
  Bottom 0.406: v21.54,40.41 v26.4,40.41
MOSI  (via drill 0.5 pad 0.3)
  Top 0.406: IC3.10 | IC3.10 v33.02,41.21 | v31.75,20.18 31.7,20.13 ISP.1
  Bottom 0.406: v33.02,41.21 32.38,41.21 31.75,40.58 v31.75,20.18
N$1
  Top 0.61: Q4.8 12.88,64.54 12.8,64.62 | Q4.7 12.62,65.81 12.6,65.84 | Q4.6 13.18,67.08 13.01,67.26 | Q4.5 12.68,68.35 12.6,68.28
  pour Top: 0,69.94 13.55,69.94 13.55,63.27 0,63.27
  pour Top: 12.93,63.7 12.93,59.14 16.19,59.14 16.19,63.7
  pour Top: 1.83,69.49 1.83,63.6 8.94,63.6 8.94,69.49
N$2
  Top 0.61: Q4.4 23.5,68.35 24.13,67.72 D3.3 26.37,66.59 R12.1
N$3
  Top 0.406: Q2.1 78.69,65.05 78.06,64.41 R9.2 | R9.2 75.51,64.54 74.24,64.54 71.24,67.55 Q1.3 | D1.C R9.2
N$4
  Top 0.406: Q1.1 R6.1
N$5
  pour Bottom: 0,80.42 0,70.57 16.19,70.57 16.19,80.42
  pour Bottom: 1.83,78.84 1.83,71.53 15.65,71.53 15.65,78.84
  pour Top: 0,80.42 0,70.57 16.19,70.57 16.19,80.42
  pour Top: 1.83,78.84 1.83,71.53 15.65,71.53 15.65,78.84
N$6
  Top 0.406: R8.1 RX_LEX.A
N$7
  Bottom 1.016: SW.4 47.52,88.8 48.79,90.07 S1.4 S1.3 S2.4 S2.3 S3.4 S3.3
N$8
  Bottom 1.016: SW.1 47.52,96.42 48.79,95.15 S1.1 S1.2
N$9
  Top 0.406: R4.2 3.66,23.7 USB_EXT.1 5.54,18.24 8.25,15.53 USB.D+
N$10
  Top 0.406: 7.64,23.27 7.62,23.27 | 7.64,23.27 7.64,23.75 R5.2 | 7.64,23.27 7.64,18.31 8.28,17.68 14.05,17.68 14.68,17.04 USB.D- 14.68,14.96 14.05,14.33 6.81,14.33 5.44,15.7 USB_EXT.2
N$11
  Top 0.406: R16.1 R17.2 35.56,64.54 34.92,63.91 34.92,61.37 34.29,60.73 R20.1
N$12
  Bottom 1.016: S2.2 S2.1 64.75,95.3 62.59,95.3 60.71,93.42 47.4,93.42 46.94,93.88 SW.2
N$13
  Bottom 1.016: S3.2 S3.1 79.85,95.1 77.83,95.1 74.47,91.75 47.24,91.75 46.84,91.34 SW.3
N$14
  Top 0.406: SJ1.3 73.34,18.82 73.98,18.19 R2.2
N$15
  Top 0.406: 80.64,19.73 Q6.1 | R24.1 80.64,19.73 | 80.64,19.73 75.98,19.73 Q5.3
N$16
  Top 0.406: C15.1 79.19,56.92 79.83,56.29 IC1.6
N$17
  Top 0.406: Q5.1 R23.1
N$18
  Top 0.406: R18.1 R19.2 arc90 56.46,66.32 IC4.3
N$19
  Top 0.406: R3.1 TX_LED.A
N$20
  Top 0.406: IC1.7 65.99,55.02 65.35,55.65 R15.2
N$21
  Top 0.406: R21.2 C18.2 arc90 53.42,60.73 57.1,60.73 57.73,61.37 IC4.2 57.73,63.91 58.37,64.54 64.72,64.54 65.35,63.91 R15.1
N$22
  Top 0.406: R27.1 R29.1 71.12,30.12 70.5,30.74 D5.3 67.31,30.74 | C20.1 66.69,30.12 67.31,30.74 | 67.31,30.74 67.31,34.7 67.94,35.33 IC5.3
N$23
  Top 0.406: Q6.3 R26.2
N$24
  Top 0.406: R33.2 R38.1 72.39,39.27 71.25,40.41 67.31,40.41 66.67,39.78 IC5.2
N$25
  Top 0.406: C21.1 59.71,51.97 60.33,51.35 D6.3 63.5,51.35 64.12,51.97 R30.1 R28.1 67.94,51.97 67.94,48.03 69.22,46.76 IC5.5
N$26
  Top 0.406: 87.81,65.45 Q3.4 81.23,66.09 Q2.2 80.59,61.69 79.96,61.05 78.69,61.05 78.05,61.05 77.42,60.41 77.42,59.14 76.78,58.51 75.51,58.51 D1.A
N$27
  Top 0.406: R34.1 R37.1 72.26,42.82 71.12,41.68 68.58,41.68 67.94,42.32 IC5.6
N$28
  Top 0.61: IC1.3 91.85,56.29 91.85,56.49 | IC1.4 91.24,57.56 91.24,57.51 | Q3.6 89.08,59 89,58.93 | Q3.7 90.35,59.05 90.22,58.93 | Q3.8 91.62,59.16 91.64,59.13 | Q3.5 87.81,58.95 87.78,58.93
  pour Top: 94.78,59.33 87.48,59.33 87.48,58.32 90.63,58.32 90.61,55.97 94.78,55.97
N$29
  Top 0.406: SJ1.1 70.8,18.82 70.17,18.19 R7.2
N$30
  Top 0.406: IC2.2 IC2.1 22.23,56.89 C3.1 21.26,56.79 20.62,56.16 L2.P$2
N$31
  Top 0.406: USB_EXT.3 10.21,13.16 11.99,11.38 13.99,11.38 14.63,12.01 14.63,13.03 USB.VBUS 16.43,13.03 17.07,13.66 17.07,23.14 16.43,23.77 11.68,23.77 R49.1
N$32
  Top 0.406: R47.1 STATUS.A
N$33
  Top 0.406: R14.1 +5V_OK.A
N$34
  Top 0.406: IC4.6 IC4.7
N$39
  Top 1.422: R52.2 C31.1
N$42  (via drill 0.5 pad 0.3)
  Top 0.406: IC5.1 v65.41,36.6 65.41,36.47 R42.2 | R38.2 v73.66,37.87
  Bottom 0.406: v65.41,36.6 73.03,36.6 73.66,37.24 v73.66,37.87
N$43  (via drill 0.5 pad 0.3)
  Top 0.406: R37.2 v73.66,44.22 | IC5.7 v66.67,45.49 66.67,45.62 R41.2
  Bottom 0.406: v66.67,45.49 73.03,45.49 73.66,44.86 v73.66,44.22
PE
  pour Top: 0,62.64 0,55.02 11.66,55.02 11.66,62.64
  pour Top: 1.63,61.77 1.63,55.27 8.33,55.27 8.33,61.77
PWM  (via drill 0.5 pad 0.3)
  Top 0.406: R1.2 69.16,58.67 R6.2 69.16,59.46 68.53,60.1 64.08,60.1 63.45,59.46 63.45,56.08 62.81,55.45 v50.41,55.45 | IC3.30 | IC3.30 v47.99,46.01
  Bottom 0.406: v47.99,46.01 49.77,46.01 50.41,46.65 v50.41,55.45
RESET  (via drill 0.5 pad 0.3)
  Top 0.406: IC3.13 | R10.1 13.97,31.94 13.34,31.3 RESET.1 | IC3.13 37.6,35.45 36.97,34.81 27.3,34.81 26.67,34.18 v26.67,31.28 26.62,31.23 ISP.5
  Bottom 0.406: RESET.1 26.67,31.3 v26.67,31.28
ROT_1
  Top 0.406: IC3.28 48.86,44.41 49.7,43.57 49.7,19.96 49.05,19.32 R40.1 49.05,14.38 49.02,14.35 C25.1
ROT_2
  Top 0.406: IC3.27 48.63,43.61 49.06,43.18 49.06,27.1 48.02,26.06 44.37,26.06 43.33,25.02 R44.1 43.33,14.38 43.31,14.35 C26.1
ROT_3
  Top 0.406: IC3.25 47.79,42.01 48.42,41.38 48.42,27.33 47.79,26.7 38.25,26.7 37.62,26.06 R46.1 37.62,14.38 37.59,14.35 C29.1
ROT_A_D+
  Bottom 1.016: 17.58,87.88 ROT.A | USB2.D+ 17.58,89.69 17.58,87.88 | 17.58,87.88 17.32,87.63 USB_ENC.1
ROT_B_D-
  Top 1.016: USB_ENC.2 10.77,90.17 13.31,87.63 16.66,87.63 | 16.66,87.63 22.02,87.63 22.66,87 ROT.B | USB2.D- 17.3,94.16 16.66,93.52 16.66,87.63
ROT_C_GND
  Bottom 1.016: ROT.C 20.12,87.99 21.34,89.2 USB2.GND 19.74,92.56 17.58,92.56 16.26,93.88 16.26,95.25 | USB_ENC.4 16.26,95.25 | ROT.SW- 16.26,97.1 16.26,95.25
ROT_EXT_1
  Top 0.406: R39.1 46.2,21.06 R40.2 46.99,17.55 47.62,16.92 47.62,11.61 46.99,10.97 45.11,10.97 44.53,10.39 ENCODER.1
ROT_EXT_2
  Top 0.406: R43.1 40.49,21.06 R44.2 41.35,17.55 41.99,16.92 ENCODER.2
ROT_EXT_3
  Top 0.406: R45.1 34.77,21.06 R46.2 35.56,17.55 36.2,16.92 36.2,12.22 36.83,11.58 38.81,11.58 39.45,10.95 ENCODER.3
ROT_SW_VBUS
  Top 1.016: USB_ENC.3 10.77,92.71 13.89,95.83 21.34,95.83 | 21.34,95.83 22.66,97.16 ROT.SW+ | USB2.VBUS 21.34,95.83
RX_LED
  Top 0.406: RX_LEX.C 4.6,39.78 5.24,39.14 17.77,39.14 21.44,42.81 IC3.8 | IC3.8
SCK
  Top 0.406: IC3.9 | IC3.9 24.77,42.01 24.08,41.33 ISP.7
SCL  (via drill 0.5 pad 0.3)
  Top 0.406: v70.17,15.01 R7.1 68.9,13.59 68.26,12.95 I2C.4 | IC3.18 v41.6,37.21 | v41.6,37.21
  Bottom 0.406: v41.6,37.21 41.6,15.65 42.24,15.01 v70.17,15.01
SDA  (via drill 0.5 pad 0.3)
  Top 0.406: IC3.19 v42.41,36.41 | v42.41,36.41 | v73.98,15.01 R2.1 72.57,13.59 71.93,12.95 71.93,11.58 70.8,10.45 I2C.3
  Bottom 0.406: v42.41,36.41 44.97,36.41 45.61,35.78 45.61,17.04 46.24,16.41 73.34,16.41 73.98,15.77 v73.98,15.01
SENSOR_1
  Top 0.406: SOLDER_IRON.4 83.77,32.16 83.13,32.79 83.13,48.54 82.5,49.17 C19.1 R25.2 R28.2
SENSOR_2  (via drill 0.5 pad 0.3)
  Top 0.406: SOLDER_IRON.2 84.45,27.08 R26.1 84.45,29.38 81.04,32.79 v80.01,32.79 77.47,32.79 R27.2 | v80.01,53.21 80.01,53.38 79.38,54.01 43.69,54.01 41.6,51.93 IC3.38
  Bottom 0.406: v80.01,53.21 v80.01,32.79
STAND
  Top 0.406: R23.2 73.03,27.21 R22.2 61.7,27.23 61.06,27.86 61.06,33.12 59.84,34.34 52.27,34.34 51.6,35.01 51.6,44.64 48.63,47.61 IC3.32
SW_1  (via drill 0.5 pad 0.3)
  Top 0.406: C30.1 66.17,17.53 R51.1 66.45,17.81 v66.45,24.99 | v48.02,42.84 47.99,42.81 IC3.26
  Bottom 0.406: v66.45,24.99 51.84,24.99 51.21,25.63 51.21,42.18 50.57,42.81 48.04,42.81 v48.02,42.84
SW_2
  Top 0.406: IC3.31 48.5,46.81 50.97,44.35 50.97,34.78 52.01,33.74 59.64,33.74 60.48,32.91 R32.1 60.48,14.38 60.45,14.35 C22.1
SW_3
  Top 0.406: C24.1 54.74,17.55 | 54.74,17.55 R36.1 | 54.74,17.55 54.74,32.47 54.1,33.11 51.78,33.11 50.33,34.56 50.33,43.97 49.09,45.21 IC3.29
SW_EXT_1
  Top 0.406: R50.1 63.35,21.06 R51.2 64.14,17.55 64.77,16.92 64.77,11.61 64.14,10.97 59.08,10.97 58.45,10.34 SWITCHES.1
SW_EXT_2
  Top 0.406: R31.1 57.63,21.06 R32.2 58.65,17.55 59.13,17.07 59.13,12.45 57.89,11.2 56.54,11.2 55.91,10.57 SWITCHES.2
SW_EXT_3
  Top 0.406: R35.1 51.92,21.06 R36.2 52.73,17.55 53.37,16.92 SWITCHES.3
T_COMP_ADC
  Top 0.406: R41.1 56.33,42.82 | 56.33,42.82 C28.1 | IC3.37 42.41,51.77 44.08,53.44 55.69,53.44 56.33,52.81 56.33,42.82
T_HEATER_ADC
  Top 0.406: R42.1 C27.1 53.44,39.27 52.81,39.91 52.81,52.2 52.17,52.83 44.3,52.83 43.2,51.74 IC3.36
TX_LED  (via drill 0.5 pad 0.3)
  Top 0.406: 4.45,44.86 TX_LED.C 3.17,44.86 2.54,44.22 2.54,39.14 3.17,38.51 v19.28,38.51 | IC3.22 v44.8,37.21 v44.81,37.21 | v25.72,38.51 v35.56,38.51
  Bottom 0.406: v19.28,38.51 v25.72,38.51 | v35.56,38.51 44.17,38.51 44.81,37.87 v44.81,37.21
U_IN_ADC
  Top 0.406: C17.1 R20.2 36.2,60.73 36.2,57.56 D4.3 39.37,57.56 40.01,56.92 IC3.40
UCAP  (via drill 0.5 pad 0.25)
  Top 0.406: IC3.6 v37.69,44.4
  Bottom 0.406: v37.69,44.4 37.72,44.42 C5.1
UVCC  (via drill 0.5 pad 0.3)
  Top 0.406: IC3.2 | R49.2 20.17,26.59 20.93,27.36 20.93,38.2 20.6,38.53 v20.6,39.61 20.83,39.59 | IC3.2 | IC3.2 v33.6,47.61 | IC3.7 | IC3.7 v36.8,43.61
  Bottom 0.406: v36.8,43.61 34.24,43.61 33.6,44.25 v33.6,47.61 33.6,47.78 32.97,48.41 21.44,48.41 20.6,47.57 v20.6,39.61
XTAL1
  Top 0.406: C8.2 45.85,32.79 45.22,33.43 Y1.2 41.44,33.43 40.8,34.06 IC3.17
XTAL2
  Top 0.406: C9.2 36.38,32.79 37.02,33.43 Y1.1 39.37,33.43 40.01,34.06 IC3.16

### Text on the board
tPlace: S1 | GND | S2 | VUSB | SW | S3 | D- | B | GND | D+ | A | WMPR / SOLDER / STATION | 1 | 1 | 5 | 4 | 1 | 7 | 2 | 1 | 1 | 1 | 6 | 03/2015

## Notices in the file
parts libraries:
SparkFun-DigitalIC: Licensing: Creative Commons ShareAlike 4.0 International - https://creativecommons.org/licenses/by-sa/4.0
